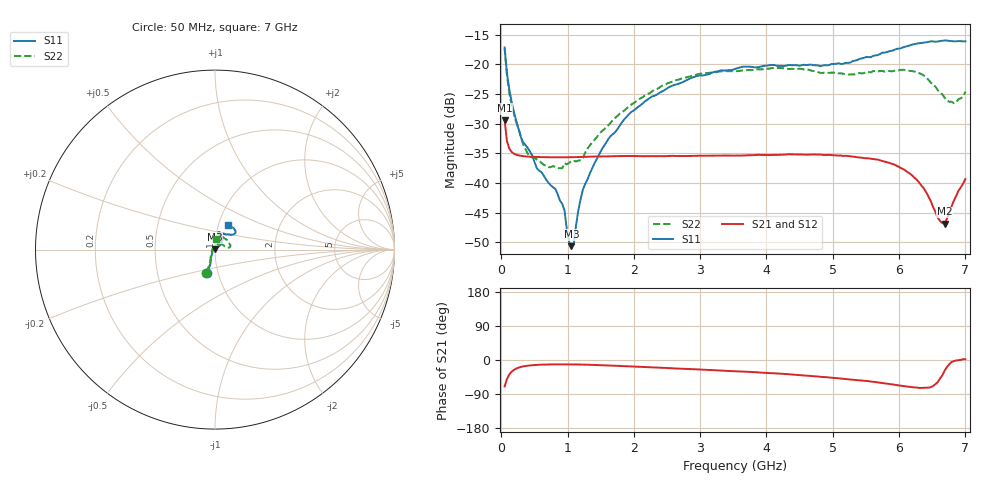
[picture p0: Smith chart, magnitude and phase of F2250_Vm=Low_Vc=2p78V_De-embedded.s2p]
! Integrated Device Technology
! Corporate Headquarters
! 6024 Silver Creek Valley Road
! San Jose, CA 95138  USA
! Phone:  1-408-284-8200
! Toll Free:  1-800-223-1366
! Webpage:  http://www.idt.com/
! Timing and RF Division
! 515 Groton Road, Suite 102
! Westford, MA 01886-6024
! Device:  F2250
! Description: Voltage Variable RF Attenuator
! Frequency:  50.0 -  6000.00 MHz
! Package:  3x3 mm Thin QFN Plastic Package: 16 pin
! Ports:  2 RF, 3 DC
!  Pin  1  = GND
!  Pin  2  = NC
!  Pin  3  = RF1  = Port 1
!  Pin  4  = NC
!  Pin  5  = GND
!  Pin  6  = GND
!  Pin  7  = GND
!  Pin  8  = GND
!  Pin  9  = NC
!  Pin 10  = RF2  = Port 2
!  Pin 11  = NC
!  Pin 12  = GND
!  Pin 13  = GND
!  Pin 14  = VCNTRL
!  Pin 15  = VDD
!  Pin 16  = VMODE
! Vcntrl:  2.780 Volts
! Vmode:  +0.000 Volts
! Vdd:  +3.30  Volts
! Current:  1.177 mA
! Data:  The device was measured on a the F2250 evaluation board which has
!  individual transmission lines to the RF pins.  Data was collected
!  using a calibrated network analyzer.  The evaluation board was
!  de-embedded using a TRL calibration technique.
!  The reference plane is the edge of the package pin.
! Misc:  SN 10
!  Action Tracker AT0258
! Date Measured:  2014-11-26
! Date:  2015-10-15  MJV
! Note:
!  Integrated Device Technology supplies this data as a sample of measured
!  data at the package pin for this product.  Your particular data for this
!  product may vary.
!  Data was taken at 25 degrees C.
!  Integrated Device Technology reserves the right to change this data at anytime.
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# GHz S dB R 50
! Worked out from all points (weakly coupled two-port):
!   201 points, 50 MHz to 7 GHz, reference 50 ohm
!   highest |S21| = -29.42 dB at 50 MHz (marker M1); lowest = -46.9 dB at 6.687 GHz (marker M2)
!   lowest |S11| = -50.7 dB at 1.058 GHz (marker M3), VSWR 1.01, Z = 49.8 + j0.243 ohm
!   |S11| at or under -10 dB: start of sweep to end of sweep
!   |S22| runs from -37.5 to -17.3 dB; largest |S21 - S12| = 5.1e-05
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0.05  -17.18 -108.6  -29.42 -69.8  -29.41 -69.8  -17.28 -111.0
0.08475  -21.45 -107.5  -32.92 -50.4  -32.92 -50.3  -21.75 -110.2
0.15425  -26.23 -116.6  -34.76 -31.1  -34.76 -31.1  -26.81 -122.4
0.29325  -32.21 -127.8  -35.43 -18.5  -35.43 -18.5  -32.09 -137.4
0.3975  -34.10 -141.9  -35.56 -15.0  -35.56 -15.0  -35.04 -160.5
0.91875  -43.52 157.8  -35.68 -11.5  -35.68 -11.5  -37.53 133.5
0.9535  -44.63 169.8  -35.68 -11.5  -35.68 -11.5  -36.66 131.2
1.023  -49.98 143.9  -35.68 -11.6  -35.67 -11.6  -36.63 115.9
1.05775  -50.66 123.7  -35.66 -11.6  -35.67 -11.6  -36.28 110.8
1.0925  -50.42 89.3  -35.66 -11.7  -35.66 -11.7  -36.30 106.4
1.162  -44.65 56.9  -35.64 -11.9  -35.64 -11.9  -36.23 95.4
1.2315  -41.09 44.2  -35.61 -12.1  -35.61 -12.1  -35.80 86.0
1.6485  -32.11 42.0  -35.52 -14.6  -35.52 -14.6  -29.87 64.5
1.96125  -28.05 42.2  -35.46 -17.2  -35.46 -17.2  -26.81 56.8
2.37825  -24.87 47.3  -35.48 -20.3  -35.48 -20.3  -23.99 56.8
3.525  -20.79 72.5  -35.40 -29.5  -35.41 -29.5  -21.19 74.7
4.7065  -20.17 72.3  -35.20 -42.6  -35.20 -42.6  -21.14 72.3
5.85325  -17.81 40.5  -36.64 -63.3  -36.63 -63.4  -21.14 23.1
6.27025  -16.51 40.0  -39.49 -72.7  -39.51 -72.8  -21.36 9.7
6.68725  -15.99 48.8  -46.86 -27.9  -46.84 -27.4  -25.63 28.6
6.861  -16.13 55.1  -42.18 -1.2  -42.15 -1.4  -26.46 57.9
7  -16.13 63.2  -39.36 1.9  -39.32 1.8  -24.63 83.1
